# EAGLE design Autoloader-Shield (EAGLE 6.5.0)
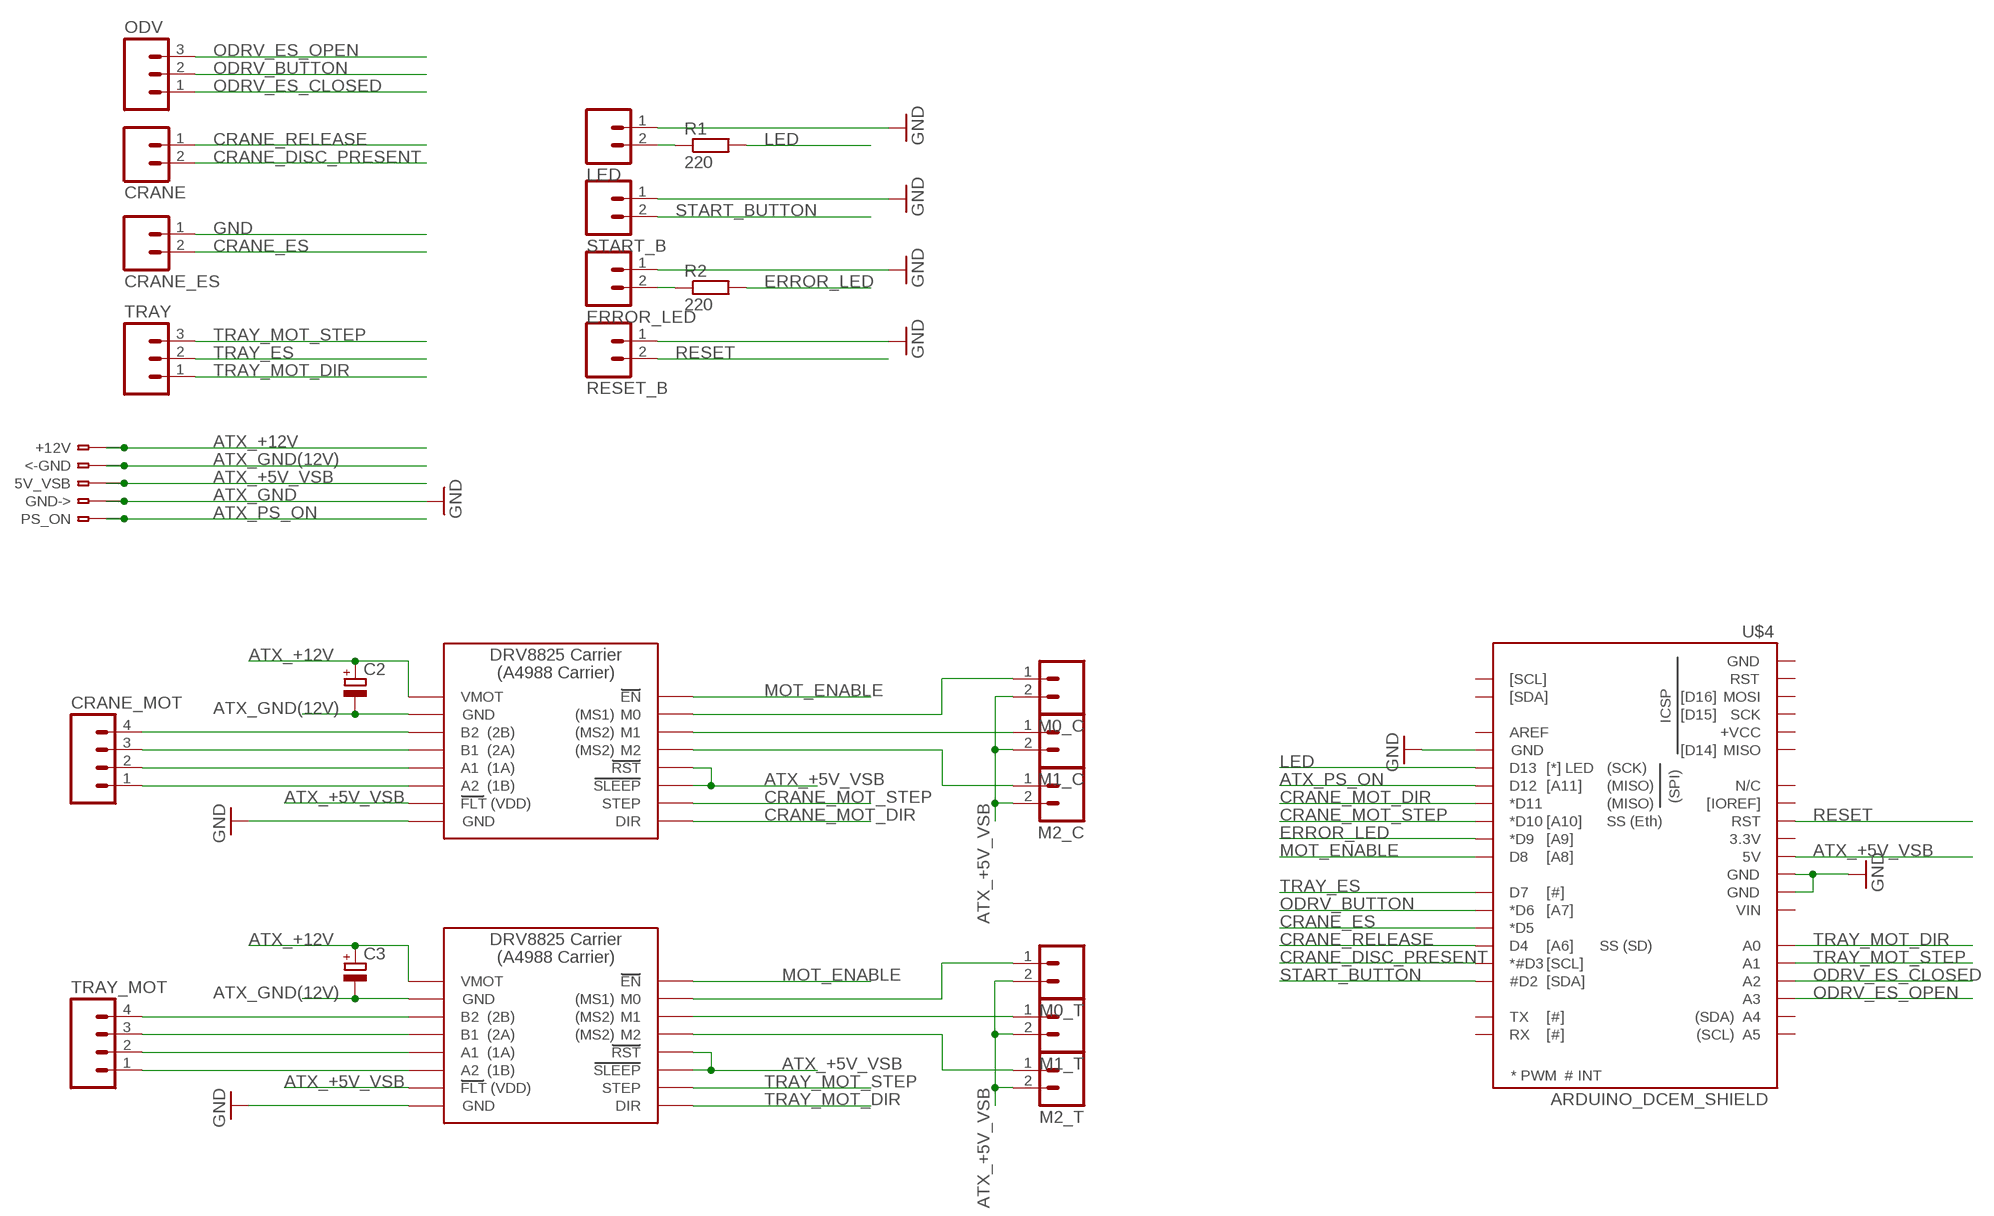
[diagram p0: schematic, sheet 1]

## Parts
5V_VSB  CON_WAGO_256-401  [CON_WAGO_256-401]
+12V  CON_WAGO_256-401  [CON_WAGO_256-401]
<-GND  CON_WAGO_256-401  [CON_WAGO_256-401]
C2  CPOL-EU153CLV-0605  [153CLV-0605]
C3  CPOL-EU153CLV-0605  [153CLV-0605]
CRANE  M02PTH  [1X02]
CRANE_ES  M02PTH  [1X02]
CRANE_MOT  M04PTH  [1X04]
ERROR_LED  M02PTH  [1X02]
GND->  CON_WAGO_256-401  [CON_WAGO_256-401]
LED  M02PTH  [1X02]
M0_C  M02PTH  [1X02]
M0_T  M02PTH  [1X02]
M1_C  M02PTH  [1X02]
M1_T  M02PTH  [1X02]
M2_C  M02PTH  [1X02]
M2_T  M02PTH  [1X02]
ODV  M03PTH  [1X03]
PS_ON  CON_WAGO_256-401  [CON_WAGO_256-401]
R1  220  R-EU_R0805  [R0805]
R2  220  R-EU_R0805  [R0805]
RESET_B  M02PTH  [1X02]
START_B  M02PTH  [1X02]
TRAY  M03PTH  [1X03]
TRAY_MOT  M04PTH  [1X04]
U$2  DRV8825(A4988)  [DRV8825(A4988)]
U$3  DRV8825(A4988)  [DRV8825(A4988)]
U$4  ARDUINO_DCEM_SHIELD  ARDUINO_DCEM_SHIELDNOSMD_NOOUTL  [ARDUINO_DCEM_SHIELD_NOSMD_NOOUTL]

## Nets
ATX_+5V_VSB: 5V_VSB.A1 5V_VSB.B1 M0_C.2 M0_T.2 M1_C.2 M1_T.2 M2_C.2 M2_T.2 U$2.FLT U$2.RST U$2.SLP(SLEEP) U$3.FLT U$3.RST U$3.SLP(SLEEP) U$4.5V
ATX_+12V: +12V.A1 +12V.B1 C2.+ C3.+ U$2.VMOT U$3.VMOT
ATX_GND: ERROR_LED.1 GND->.A1 GND->.B1 LED.1 RESET_B.1 START_B.1 U$2.GND@1(GND) U$3.GND@1(GND) U$4.GND0 U$4.GND1 U$4.GND@DP(GND) ; supply symbol labelled GND
ATX_GND(12V): <-GND.A1 <-GND.B1 C2.- C3.- U$2.GND@0(GND) U$3.GND@0(GND)
ATX_PS_ON: PS_ON.A1 PS_ON.B1 U$4.D12
CRANE_DISC_PRESENT: CRANE.2 U$4.D3(*#D3)
CRANE_ES: CRANE_ES.2 U$4.D5(*D5)
CRANE_MOT_DIR: U$2.DIR U$4.D11(*D11)
CRANE_MOT_M0: M0_C.1 U$2.M0
CRANE_MOT_M1: M1_C.1 U$2.M1
CRANE_MOT_M2: M2_C.1 U$2.M2
CRANE_MOT_STEP: U$2.STEP U$4.D10(*D10)
CRANE_RELEASE: CRANE.1 U$4.D4
ERROR_LED: R2.2 U$4.D9(*D9)
GND: CRANE_ES.1
LED: R1.2 U$4.D13
MOT_ENABLE: U$2.EN U$3.EN U$4.D8
N$1: TRAY_MOT.4 U$3.B2
N$3: TRAY_MOT.3 U$3.B1
N$5: TRAY_MOT.2 U$3.A1
N$6: TRAY_MOT.1 U$3.A2
N$7: CRANE_MOT.4 U$2.B2
N$8: CRANE_MOT.3 U$2.B1
N$9: CRANE_MOT.2 U$2.A1
N$10: CRANE_MOT.1 U$2.A2
N$17: ERROR_LED.2 R2.1
N$18: LED.2 R1.1
ODRV_BUTTON: ODV.2 U$4.D6(*D6)
ODRV_ES_CLOSED: ODV.1 U$4.A2
ODRV_ES_OPEN: ODV.3 U$4.A3
RESET: RESET_B.2 U$4.RST
START_BUTTON: START_B.2 U$4.D2(#D2)
TRAY_ES: TRAY.2 U$4.D7
TRAY_MOT_DIR: TRAY.1 U$3.DIR U$4.A0
TRAY_MOT_M0: M0_T.1 U$3.M0
TRAY_MOT_M1: M1_T.1 U$3.M1
TRAY_MOT_M2: M2_T.1 U$3.M2
TRAY_MOT_STEP: TRAY.3 U$3.STEP U$4.A1
Unconnected: U$4.3.3V U$4.+VCC@ICSP(+VCC) U$4.A4 U$4.A5 U$4.AREF U$4.GND@ICSP(GND) U$4.IOREF([IOREF]) U$4.MISO U$4.MOSI U$4.N/C U$4.RST@ICSP(RST) U$4.RX U$4.SCK U$4.SCL([SCL]) U$4.SDA([SDA]) U$4.TX U$4.VIN

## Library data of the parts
5V_VSB +12V <-GND GND-> PS_ON = library_1:CON_WAGO_256-401: Wago 256-401
C2 C3 = rcl:CPOL-EU: POLARIZED CAPACITOR, European symbol
CRANE CRANE_ES ERROR_LED LED M0_C M0_T M1_C M1_T M2_C M2_T RESET_B START_B = SparkFun:M02: Header 2
CRANE_MOT TRAY_MOT = SparkFun:M04: Header 4 Standard 4-pin 0.1" header. Use with straight break away headers (SKU : PRT-00116), right angle break away headers (PRT-00553), swiss pins (PRT-00743), machine pins (PRT-00117), and female headers (PRT-00115). Molex polarized connector foot print use with SKU : PRT-08231 with associated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
ODV TRAY = SparkFun:M03: Header 3 Standard 3-pin 0.1" header. Use with straight break away headers (SKU : PRT-00116), right angle break away headers (PRT-00553), swiss pins (PRT-00743), machine pins (PRT-00117), and female headers (PRT-00115). Molex polarized connector foot print use with SKU : PRT-08232 with associated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
R1 R2 = rcl:R-EU_: RESISTOR, European symbol
U$2 U$3 = library_1:DRV8825(A4988)
U$4 = library_1:ARDUINO_DCEM_SHIELD

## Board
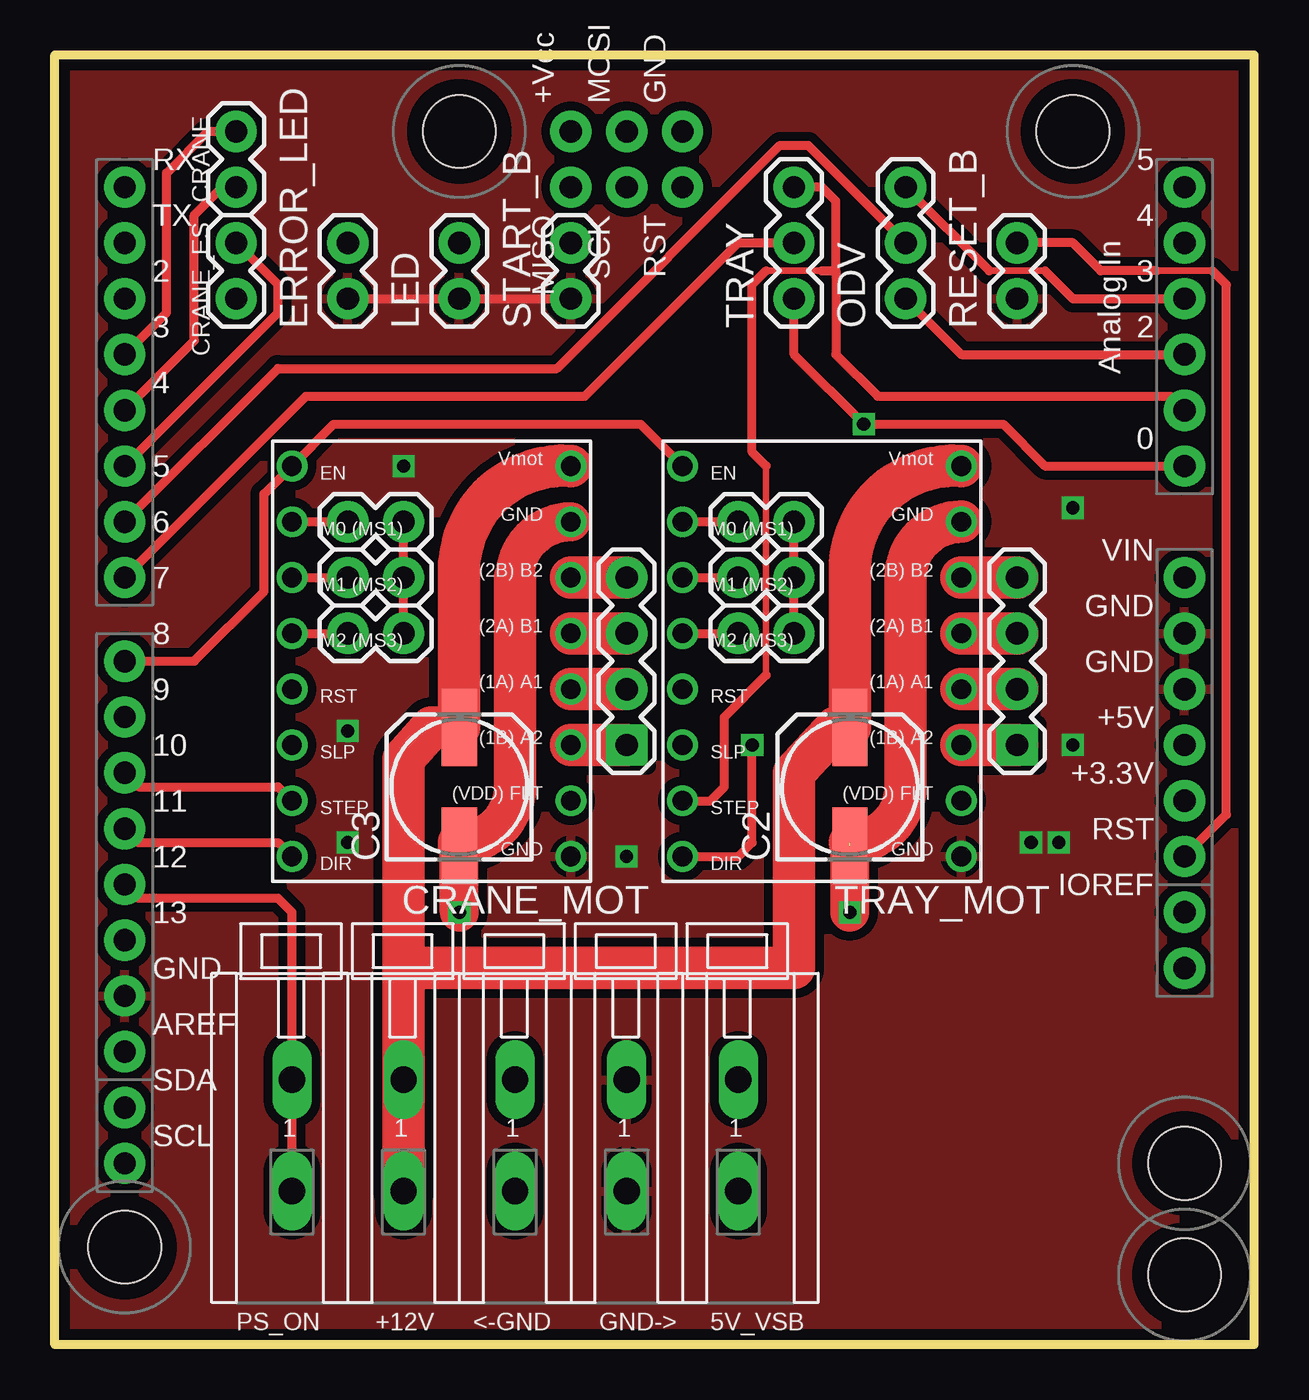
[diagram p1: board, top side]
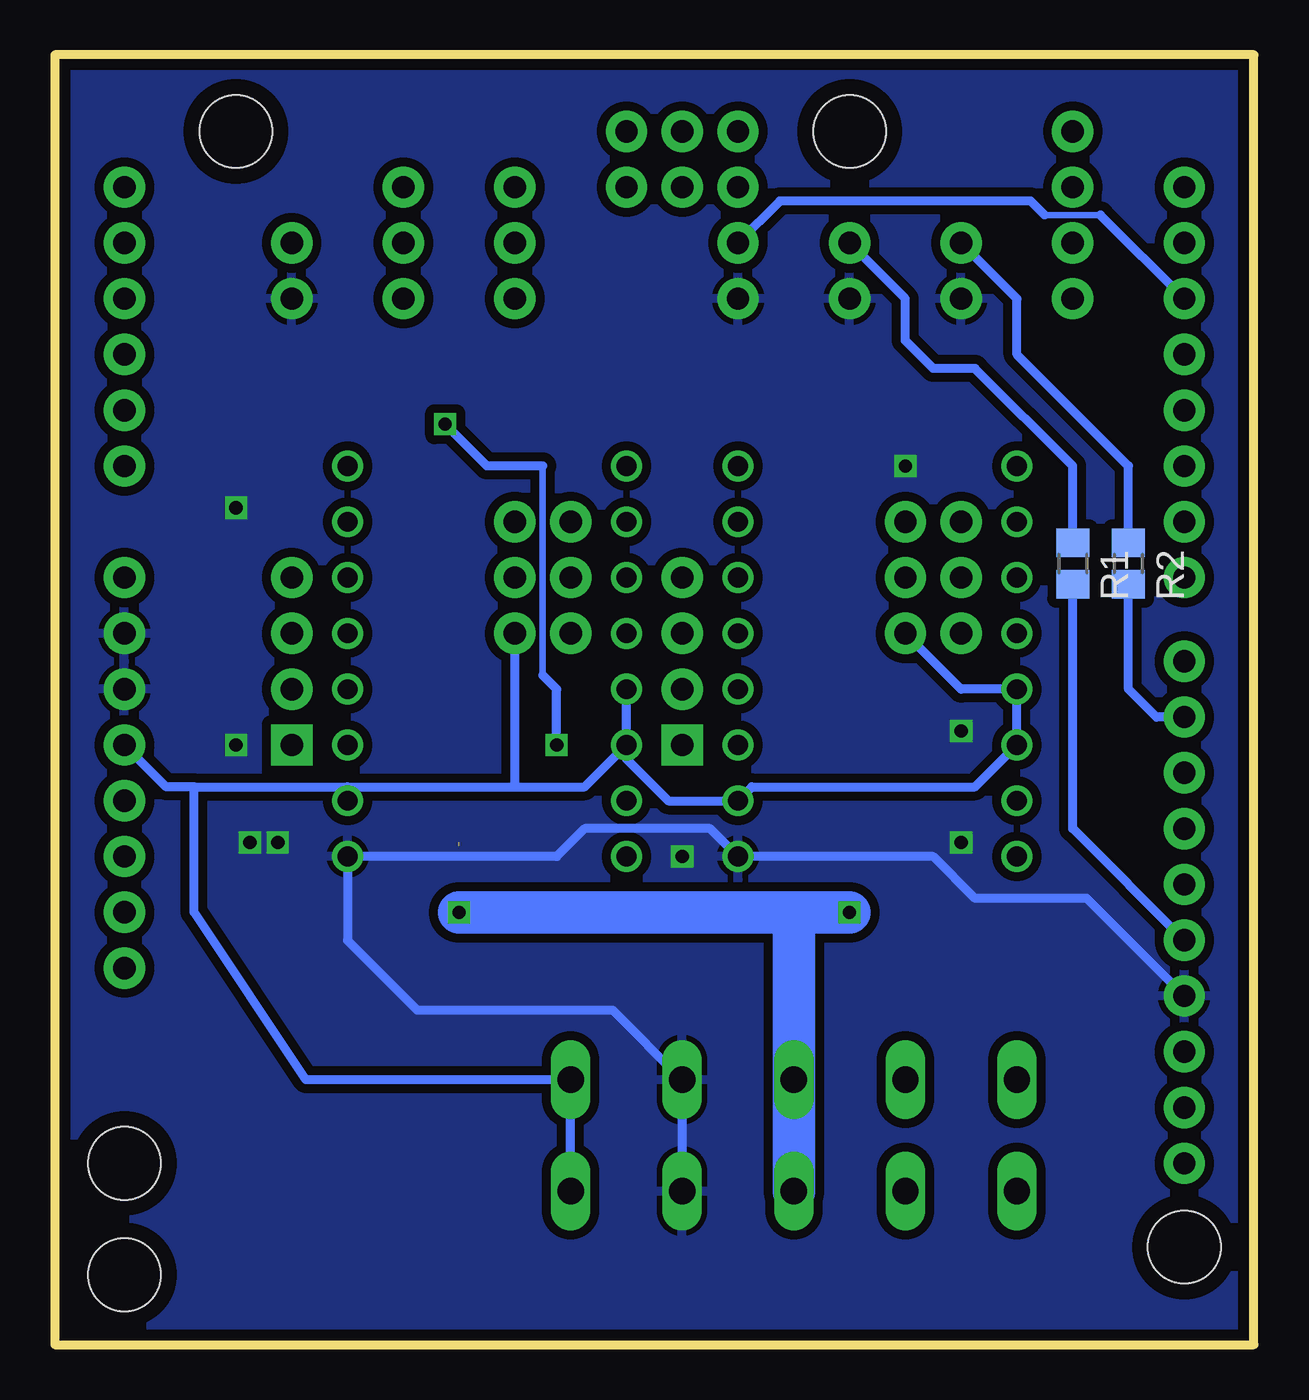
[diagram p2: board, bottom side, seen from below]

Size 54.6 x 58.72 mm. Coordinates in mm from the lower left corner, seen from the top.
Outline: 0,58.73 54.6,58.73 54.6,0 0,0 0,58.73
Copper layers (1*16): Top 0.035mm / dielectric 1.5mm / Bottom 0.035mm
Design rules "default *": minimum track width 10mil, minimum drill 12mil, track to track 6mil, track to pad 6mil, pad to pad 8mil, via to via 8mil, smd to smd 8mil, copper to edge 20mil, drill to drill 8mil, minimum pad ring 10mil, minimum via ring 8mil, stop-mask expansion 4mil, vias tented up to drill 0mil, thermal gap 10mil

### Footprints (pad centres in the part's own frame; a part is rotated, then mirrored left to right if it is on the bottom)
CON_WAGO_256-401 = drill 1.2 long: A1 2.54,10.16; B1 2.54,5.08
153CLV-0605 = smd 3.5 x 1.6: + 2.7,0; - -2.7,0
1X02 = drill 1.016 pad 1.88: 1 0,0; 2 2.54,0
1X04 = drill 1.016 pad 1.88 square: 1 0,0 | drill 1.016 pad 1.88: 2 2.54,0; 3 5.08,0; 4 7.62,0
1X03 = drill 1.016 pad 1.88: 1 0,0; 2 2.54,0; 3 5.08,0
R0805 = smd 1.3 x 1.5: 1 -0.95,0; 2 0.95,0
DRV8825(A4988) = drill 0.9: A1 13.97,8.89; A2 13.97,6.35; B1 13.97,11.43; B2 13.97,13.97; DIR 1.27,1.27; EN 1.27,19.05; FLT 13.97,3.81; GND@0 13.97,16.51; GND@1 13.97,1.27; M0 1.27,16.51; M1 1.27,13.97; M2 1.27,11.43; RST 1.27,8.89; SLP 1.27,6.35; STEP 1.27,3.81; VMOT 13.97,19.05
ARDUINO_DCEM_SHIELD_NOSMD_NOOUTL = drill 1.016 pad 1.88: 3.3V 50.8,35.56; 5V 50.8,38.1; +VCC@ICSP 22.86,66.04; A0 50.8,50.8; A1 50.8,53.34; A2 50.8,55.88; A3 50.8,58.42; A4 50.8,60.96; A5 50.8,63.5; AREF 2.54,24.13; D2 2.54,58.42; D3 2.54,55.88; D4 2.54,53.34; D5 2.54,50.8; D6 2.54,48.26; D7 2.54,45.72; D8 2.54,41.91; D9 2.54,39.37; D10 2.54,36.83; D11 2.54,34.29; D12 2.54,31.75; D13 2.54,29.21; GND0 50.8,40.64; GND1 50.8,43.18; GND@DP 2.54,26.67; GND@ICSP 27.94,66.04; IOREF 50.8,30.48; MISO 22.86,63.5; MOSI 25.4,66.04; N/C 50.8,27.94; RST 50.8,33.02; RST@ICSP 27.94,63.5; RX 2.54,63.5; SCK 25.4,63.5; SCL 2.54,19.05; SDA 2.54,21.59; TX 2.54,60.96; VIN 50.8,45.72 | hole 3.3: 45.72,66.04; 17.78,66.04; 50.8,19.05; 2.54,15.24; 50.8,13.97

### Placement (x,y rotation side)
5V_VSB  28.57,1.91 0 top
+12V  13.34,1.91 0 top
<-GND  18.41,1.91 0 top
C2  36.2,25.4 90 top
C3  18.41,25.4 90 top
CRANE  8.26,52.7 90 top
CRANE_ES  8.26,47.62 90 top
CRANE_MOT  26.04,27.3 90 top
ERROR_LED  13.34,47.62 90 top
GND->  23.5,1.91 0 top
LED  18.41,47.62 90 top
M0_C  13.34,37.47 0 top
M0_T  31.11,37.47 0 top
M1_C  13.34,34.92 0 top
M1_T  31.11,34.92 0 top
M2_C  13.34,32.38 0 top
M2_T  31.11,32.38 0 top
ODV  38.73,47.62 90 top
PS_ON  8.26,1.91 0 top
R1  8.26,35.56 270 bottom
R2  5.71,35.56 270 bottom
RESET_B  43.81,47.62 90 top
START_B  23.5,47.62 90 top
TRAY  33.66,47.62 90 top
TRAY_MOT  43.81,27.3 90 top
U$2  9.53,20.95 0 top
U$3  27.3,20.95 0 top
U$4  0.64,-10.79 0 top

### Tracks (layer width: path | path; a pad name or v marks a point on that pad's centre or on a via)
ATX_+5V_VSB
  Top 0.406: M0_T.2 M1_T.2 M2_T.2 | M0_C.2 M1_C.2 M2_C.2
  Bottom 0.406: U$3.SLP 28.57,26.67 26.67,24.77 U$2.FLT 22.86,25.4 12.7,25.4 U$2.SLP U$2.RST 13.34,29.84 M2_C.2 | U$3.SLP U$3.RST | U$3.SLP 30.48,25.4 33.66,25.4 | 41.27,25.4 33.66,25.4 | 48.26,25.4 41.27,25.4 | 48.26,25.4 49.53,25.4 U$4.5V | 41.27,25.4 U$3.FLT | 48.26,25.4 48.26,19.68 43.18,12.06 5V_VSB.A1 5V_VSB.B1 | 33.66,25.4 M2_T.2
ATX_+12V
  Top 1.93: U$3.VMOT arc90 36.2,35.56 C2.+ 35.56,28.1 33.66,26.04 33.66,17.14 15.88,17.14 | U$2.VMOT arc90 18.41,35.56 C3.+ 17.14,28.1 15.88,26.67 15.88,17.14 | +12V.B1 +12V.A1 15.88,17.14
ATX_GND  (via drill 0.6)
  Top 0.406: START_B.1 LED.1 ERROR_LED.1
  Bottom 0.406: GND->.B1 GND->.A1 29.21,15.24 38.1,15.24 41.27,18.41 U$3.GND@1 31.75,22.23 30.48,23.5 24.77,23.5 U$2.GND@1 14.61,22.23 12.7,20.32 7.62,20.32 U$4.GND@DP
  other vias: 13.34,22.86 44.45,22.86 45.72,22.86 46.35,27.3 46.35,38.1 15.88,40.01 13.34,27.94 26.04,22.23
  pour Bottom (isolate 0.406): 0,0 0,58.42 54.61,58.42 54.61,15.24 54.61,0
  pour Top (isolate 0.406): 0,0 0,58.42 54.61,58.42 54.61,0
ATX_GND(12V)  (via drill 0.6)  (1 unrouted)
  Top 1.778: 20.95,34.92 arc-90 U$2.GND@0 | v18.41,19.68 C3.- | v36.2,19.68 C2.-
  Top 1.93: U$3.GND@0 arc90 38.73,34.92 38.73,25.4 arc-90 36.2,22.86 | 20.95,34.92 20.95,25.4 arc-90 18.41,22.86 C3.-
  Bottom 1.93: 20.95,19.68 v18.41,19.68 | 20.95,19.68 v36.2,19.68 | <-GND.B1 <-GND.A1 20.95,19.68
ATX_PS_ON
  Top 0.406: U$4.D12 3.81,20.32 10.16,20.32 10.79,19.68 PS_ON.A1 PS_ON.B1
CRANE_DISC_PRESENT
  Top 0.406: U$4.D3 5.08,46.99 5.08,53.34 6.99,55.24 CRANE.2
CRANE_ES
  Top 0.406: U$4.D5 10.16,46.99 10.16,48.26 CRANE_ES.2
CRANE_MOT_DIR
  Top 0.406: U$4.D11 3.81,22.86 10.16,22.86 U$2.DIR
CRANE_MOT_M0
  Top 0.406: U$2.M0 M0_C.1
CRANE_MOT_M1
  Top 0.406: U$2.M1 M1_C.1
CRANE_MOT_M2
  Top 0.406: U$2.M2 M2_C.1
CRANE_MOT_STEP
  Top 0.406: U$4.D10 3.81,25.4 10.16,25.4 U$2.STEP
CRANE_RELEASE
  Top 0.406: U$4.D4 6.35,45.72 6.35,51.44 7.62,52.7 CRANE.1
ERROR_LED
  Bottom 0.406: U$4.D9 4.45,28.57 5.71,29.84 R2.2
LED
  Bottom 0.406: U$4.D13 8.26,23.5 R1.2
MOT_ENABLE
  Top 0.406: U$3.EN 26.67,41.91 12.7,41.91 U$2.EN 9.53,38.73 9.53,34.29 6.35,31.11 U$4.D8
N$1
  Top 1.93: U$3.B2 TRAY_MOT.4
N$3
  Top 1.93: U$3.B1 TRAY_MOT.3
N$5
  Top 1.93: U$3.A1 TRAY_MOT.2
N$6
  Top 1.93: U$3.A2 TRAY_MOT.1
N$7
  Top 1.93: U$2.B2 CRANE_MOT.4
N$8
  Top 1.93: U$2.B1 CRANE_MOT.3
N$9
  Top 1.93: U$2.A1 CRANE_MOT.2
N$10
  Top 1.93: U$2.A2 CRANE_MOT.1
N$17
  Bottom 0.406: R2.1 5.71,40.01 10.79,45.09 10.79,47.62 ERROR_LED.2
N$18
  Bottom 0.406: R1.1 8.26,40.01 12.7,44.45 14.61,44.45 15.88,45.72 15.88,47.62 LED.2
ODRV_BUTTON
  Top 0.406: ODV.2 34.29,54.61 33.02,54.61 22.86,44.45 10.16,44.45 U$4.D6
ODRV_ES_CLOSED
  Top 0.406: U$4.A2 41.27,45.09 ODV.1
ODRV_ES_OPEN
  Top 0.305: 42.55,48.9 45.09,48.9
  Top 0.406: ODV.3 42.55,48.9 | 45.09,48.9 46.35,47.62 U$4.A3
RESET
  Top 0.305: 52.7,48.9 50.16,48.9
  Top 0.406: U$4.RST 53.34,24.13 53.34,48.26 52.7,48.9 | RESET_B.2 46.35,50.16 47.62,48.9 50.16,48.9
START_BUTTON
  Bottom 0.305: 6.99,51.44 9.53,51.44
  Bottom 0.406: U$4.D2 6.99,51.44 | START_B.2 21.59,52.07 10.16,52.07 9.53,51.44
TRAY_ES
  Top 0.406: U$4.D7 11.43,43.18 24.13,43.18 31.11,50.16 TRAY.2
TRAY_MOT_DIR  (via drill 0.6)
  Top 0.406: U$3.DIR 31.11,22.23 31.75,22.86 v31.75,27.3 | U$4.A0 45.09,40.01 43.18,41.91 v36.83,41.91 33.66,45.09 TRAY.1
  Bottom 0.305: 32.38,30.48 32.38,40.01
  Bottom 0.406: v31.75,27.3 31.75,29.84 32.38,30.48 | 32.38,40.01 34.92,40.01 v36.83,41.91
TRAY_MOT_M0
  Top 0.406: U$3.M0 M0_T.1
TRAY_MOT_M1
  Top 0.406: U$3.M1 M1_T.1
TRAY_MOT_M2
  Top 0.406: U$3.M2 M2_T.1
TRAY_MOT_STEP
  Top 0.305: 32.38,30.48 32.38,40.01 | 32.38,48.9 34.92,48.9
  Top 0.406: U$3.STEP 29.84,24.77 30.48,25.4 30.48,28.57 32.38,30.48 | TRAY.3 34.92,52.7 35.56,52.07 35.56,48.9 | U$4.A1 50.8,43.18 37.47,43.18 35.56,45.09 35.56,48.9 | 32.38,40.01 31.75,40.64 31.75,48.26 32.38,48.9 | 34.92,48.9 35.56,48.9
